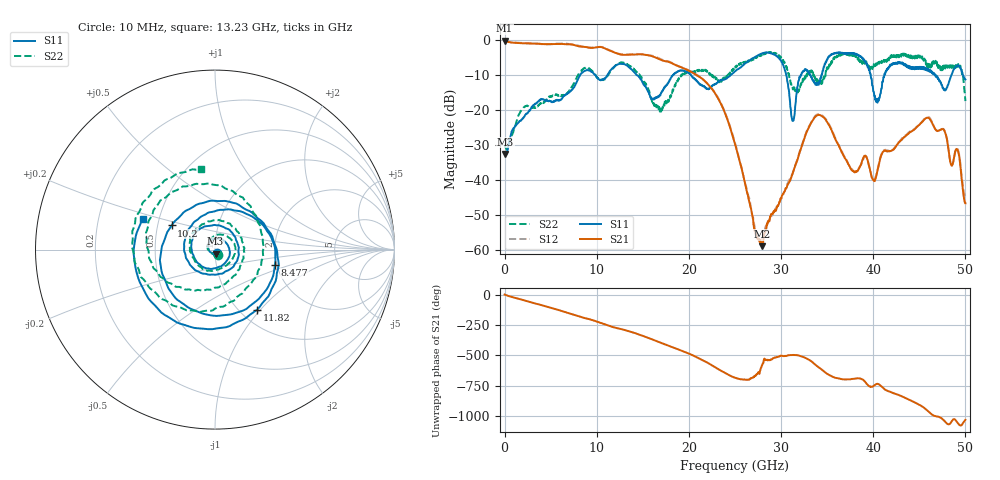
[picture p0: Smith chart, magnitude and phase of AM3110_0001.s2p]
# Hz S DB R 50.0
!freq dBS11 angS11 dBS21 angS21 dBS12 angS12 dBS22 angS22
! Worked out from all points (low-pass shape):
!   1601 points, 10 MHz to 50 GHz, reference 50 ohm
!   highest |S21| = -0.17 dB at 10 MHz (marker M1); lowest = -59.0 dB at 27.91 GHz (marker M2)
!   |S21| within 3 dB of the highest: start of sweep to 11.59 GHz
!   lowest |S11| = -32.6 dB at 103.7 MHz (marker M3), VSWR 1.05, Z = 50.2 - j2.33 ohm
!   |S11| at or under -10 dB: start of sweep to 8.203 GHz; 14.34 GHz to 18.27 GHz (3.931 GHz wide, 24.1 % of centre); 20.23 GHz to 24.54 GHz (4.309 GHz wide, 19.2 % of centre)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
!   |S22| runs from -31.4 to -3.4 dB; largest |S21 - S12| = 0.026
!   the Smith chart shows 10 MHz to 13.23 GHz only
!   S11 on the Smith chart (normalised r, x): 10 MHz: 1.02, -0.04; 8.477 GHz: 1.96, -0.38; 10.2 GHz: 0.59, +0.17; 11.82 GHz: 1.19, -0.96; 13.23 GHz: 0.40, +0.17
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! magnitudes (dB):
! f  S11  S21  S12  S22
! 10 MHz  -32.5  -0.2  -0.1  -29.9
! 103.7 MHz  -32.6  -0.2  -0.1  -30.7
! 8.352 GHz  -9.5  -1.9  -1.7  -8.6
! 8.477 GHz  -9.2  -1.9  -1.7  -8.3
! 10.2 GHz  -11.2  -1.9  -1.9  -11.1
! 11.82 GHz  -7.8  -3.4  -3.3  -7.9
! 13.23 GHz  -7.2  -4.2  -4.1  -6.9
! 16.69 GHz  -16.2  -5.3  -5.1  -19.0
! 19.04 GHz  -8.7  -7.6  -7.6  -10.7
! 21.97 GHz  -13.9  -12.4  -12.3  -9.1
! 25 GHz  -8.9  -29.8  -29.4  -7.9
! 27.91 GHz  -3.8  -59.0  -56.7  -4.2
! 30.13 GHz  -6.5  -44.5  -44.9  -5.3
! 31.25 GHz  -23.1  -38.2  -38.0  -13.7
! 32.16 GHz  -10.1  -31.1  -30.7  -12.6
! 33.35 GHz  -10.8  -23.4  -23.2  -8.8
! 37.88 GHz  -3.7  -37.7  -37.6  -4.1
! 40.03 GHz  -14.7  -40.1  -40.1  -7.6
! 41.69 GHz  -7.8  -31.8  -31.7  -5.8
! 46.03 GHz  -8.7  -22.3  -22.1  -6.9
! 49.16 GHz  -7.2  -31.5  -31.2  -7.6
! 50 GHz  -11.3  -46.8  -44.4  -17.5
